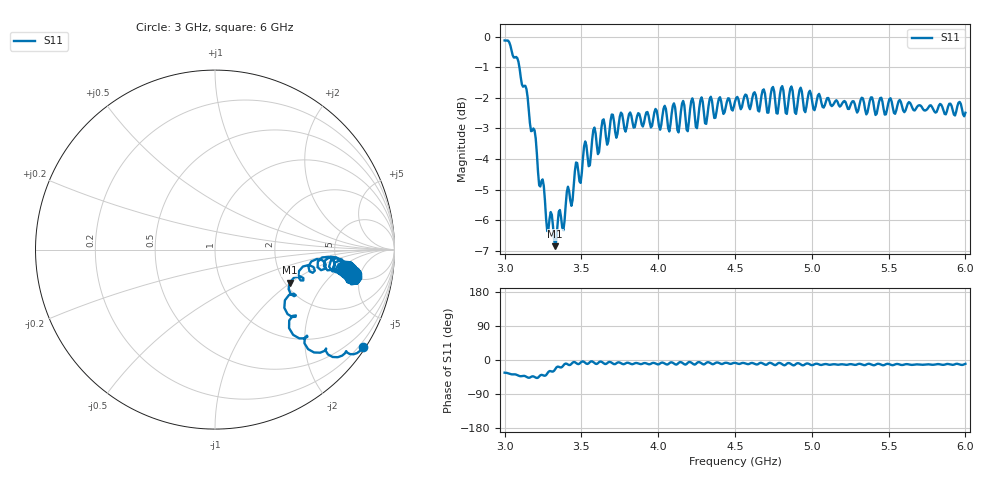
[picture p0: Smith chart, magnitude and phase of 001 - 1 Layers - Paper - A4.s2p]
!  02/07/2025  14:32:19
! Ref Plane: 0.000 mm
# MHZ S MA R  50
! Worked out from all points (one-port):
!   401 points, 3 GHz to 6 GHz, reference 50 ohm
!   lowest |S11| = -6.8 dB at 3.33 GHz (marker M1), VSWR 2.67, Z = 106 - j49 ohm
!   |S11| at or under -10 dB: nowhere
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3000  0.9855 -33.5
3090  0.9098 -41.2
3150  0.7957 -46.1
3217.5  0.6014 -46.7
3330  0.4547 -23.9
3375  0.4881 -18.1
3450  0.5705 -5.3
3525  0.6742 -7.5
3750  0.7402 -6.8
4102.5  0.778 -9.3
4125  0.7032 -10.8
4155  0.7771 -6.9
4192.5  0.7006 -7.4
4215  0.7844 -6.8
4252.5  0.7086 -7.6
4275  0.7876 -6.9
4500  0.783 -7.7
4725  0.7762 -7.4
4755  0.814 -12.8
4792.5  0.8046 -7.9
4815  0.8166 -13.2
4852.5  0.8017 -8.2
4875  0.8159 -13.4
4912.5  0.7966 -8.5
4942.5  0.7857 -14.1
5250  0.7702 -10.9
5625  0.7773 -11.2
6000  0.7509 -10.1
